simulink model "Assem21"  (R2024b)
settings: Solver=VariableStepAuto  StartTime=0.0  StopTime=5.0  RelTol=1e-3
model workspace: external: MATLAB File (data not in the file)
undefined symbols (not defined in the file or in its folder): deg, kg, Levenberg, m, Marquardt, mm, N, s, smiData, X, Y, Z
libraries: sm_lib x57, nesl_utility x7, robotcorelib x3, robotmaniplib x2
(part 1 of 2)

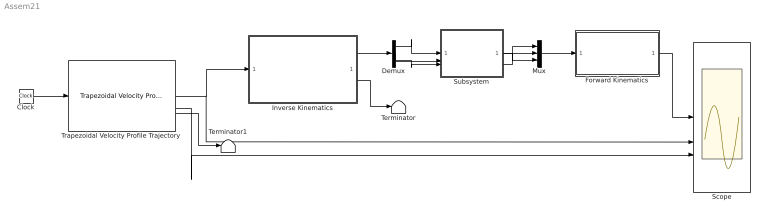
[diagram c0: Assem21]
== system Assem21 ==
  Clock : Clock
  Demux : Demux  Outputs=3
  Forward Kinematics : Subsystem
  Inverse Kinematics : Subsystem
  Mux : Mux  Inputs=3
  Scope : Scope  NumInputPorts=3
  Subsystem : Subsystem
  Terminator : Terminator
  Terminator1 : Terminator
  Trapezoidal Velocity Profile Trajectory : robotcorelib/Trapezoidal Velocity Profile Trajectory  WaypointSource=Internal  Waypoints=wp  NumParams=1  Parameter1=End Time  Parameter2=End Time  ParameterSource=Internal  PeakVelocity=[ 2; 2 ]  Acceleration=[ 1; 2 ]  EndTime=[0.5 1 1 0.5 0.5;0.5 1 1 0.5 0.5;0.5 1 1 0.5 0.5]  AccelTime=[ 1; 2 ]  SimulateUsing=Interpreted execution
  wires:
  Subsystem/2(q2m) -> Mux/2
  Subsystem/1(q1m) -> Mux/1
  Subsystem/3(q3m) -> Mux/3
  Mux/1 -> Forward Kinematics/1(Config)
  Demux/1 -> Subsystem/1(q1)
  Demux/2 -> Subsystem/2(q2)
  Demux/3 -> Subsystem/3(q3)
  Forward Kinematics/1(XYX EE) -> Scope/1
  Inverse Kinematics/1(Config) -> Demux/1
  Inverse Kinematics/2(Info) -> Terminator/1
  Clock/1 -> Trapezoidal Velocity Profile Trajectory/1
  Trapezoidal Velocity Profile Trajectory/1 -> Scope/2, Inverse Kinematics/1(In1)
  Trapezoidal Velocity Profile Trajectory/3 -> Terminator1/1
  Trapezoidal Velocity Profile Trajectory/2 -> Scope/3

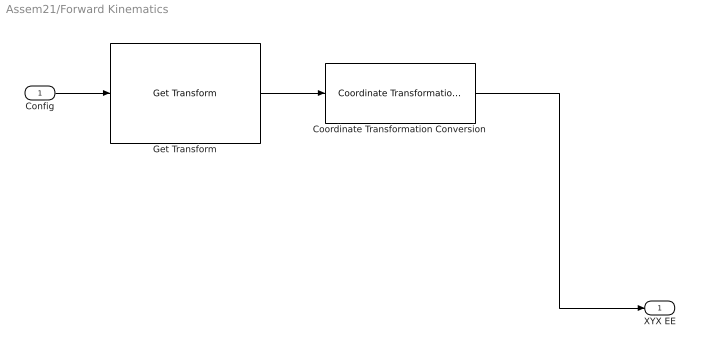
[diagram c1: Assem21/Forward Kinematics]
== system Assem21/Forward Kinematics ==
  Config : Inport
  Coordinate Transformation Conversion : robotcorelib/Coordinate Transformation Conversion  InputRepresentation=Homogeneous Transformation  InputEulerSequence=ZYX  ShowTrVecInputPort=on  OutputRepresentation=Translation Vector  OutputEulerSequence=ZYX  ShowTrVecOutputPort=on  SimulateUsing=Interpreted execution
  Get Transform : robotmaniplib/Get Transform  RigidBodyTree=DOF3_Arm  SourceBody=Body3  TargetBody=Base  SimulateUsing=Interpreted execution
  XYX EE : Outport
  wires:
  Get Transform/1 -> Coordinate Transformation Conversion/1
  Config/1 -> Get Transform/1
  Coordinate Transformation Conversion/1 -> XYX EE/1

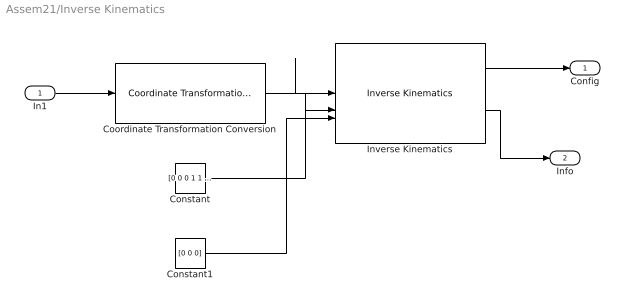
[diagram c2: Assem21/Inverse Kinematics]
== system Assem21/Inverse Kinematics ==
  In1 : Inport
  Constant : Constant  Value=[0 0 0 1 1 1]
  Constant1 : Constant  Value=[0 0 0]
  Coordinate Transformation Conversion : robotcorelib/Coordinate Transformation Conversion  InputRepresentation=Translation Vector  InputEulerSequence=ZYX  ShowTrVecInputPort=on  OutputRepresentation=Homogeneous Transformation  OutputEulerSequence=ZYX  ShowTrVecOutputPort=on  SimulateUsing=Interpreted execution
  Inverse Kinematics : robotmaniplib/Inverse Kinematics  RigidBodyTree=DOF3_Arm  EndEffector=Body3  ShowInfo=on  SolverName=Levenberg-Marquardt  EnforceJointLimits=on  MaxIterations=1500  MaxTime=10  GradientTolerance=1e-3  SolutionTolerance=1e-2  StepTolerance=1e-14  ErrorChangeTolerance=1e-3  UseErrorDamping=on  DampingBias=0.0025  SimulateUsing=Interpreted execution
  Config : Outport
  Info : Outport  Port=2
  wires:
  Constant/1 -> Inverse Kinematics/2
  In1/1 -> Coordinate Transformation Conversion/1
  Coordinate Transformation Conversion/1 -> Inverse Kinematics/1
  Inverse Kinematics/2 -> Info/1
  Inverse Kinematics/1 -> Config/1
  Constant1/1 -> Inverse Kinematics/3

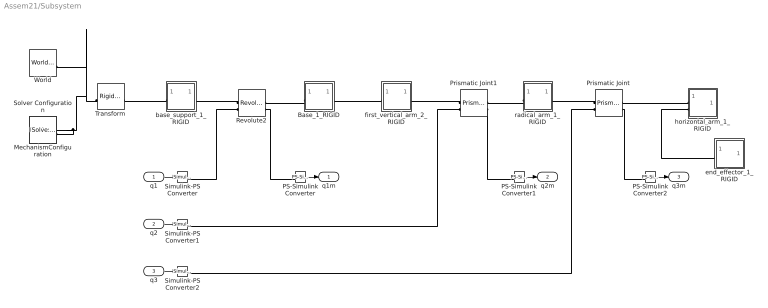
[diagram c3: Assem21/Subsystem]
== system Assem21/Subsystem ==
  q1 : Inport
  q2 : Inport  Port=2
  q3 : Inport  Port=3
  Base_1_RIGID : Subsystem
  MechanismConfiguration : sm_lib/Utilities/Mechanism Configuration  UniformGravity=Constant  GravityVector=[0 -9.80665 0]  GravityVectorUnits=m/s^2  LinearizationDelta=0.001  JointModeTransitionNonlinearIterations=2
  PS-Simulink Converter : nesl_utility/PS-Simulink Converter  PhysicalDomain=network_engine_domain  SubClassName=ps_output  LeftPortType=input  RightPortType=output  PseudoPeriodic=off  Frequencies=[]  VectorFormat=inherit  Unit=inherit  AffineConversion=off
  PS-Simulink Converter1 : nesl_utility/PS-Simulink Converter  PhysicalDomain=network_engine_domain  SubClassName=ps_output  LeftPortType=input  RightPortType=output  PseudoPeriodic=off  Frequencies=[]  VectorFormat=inherit  Unit=inherit  AffineConversion=off
  PS-Simulink Converter2 : nesl_utility/PS-Simulink Converter  PhysicalDomain=network_engine_domain  SubClassName=ps_output  LeftPortType=input  RightPortType=output  PseudoPeriodic=off  Frequencies=[]  VectorFormat=inherit  Unit=inherit  AffineConversion=off
  Prismatic Joint : sm_lib/Joints/Prismatic Joint  JointMode=Normal  CompositeWrenchDir=FollowerOnBase  CompositeWrenchFrame=BaseFrame  SenseConstraintForce=off  SenseConstraintTorque=off  SenseTotalForce=off  SenseTotalTorque=off  PositionTargetSpecify=off  PositionTargetPriority=High  PositionTargetValue=0  PositionTargetValueUnits=m  VelocityTargetSpecify=off  VelocityTargetPriority=High  VelocityTargetValue=0  VelocityTargetValueUnits=m/s  EquilibriumPosition=0  EquilibriumPositionUnits=m  SpringStiffness=0  SpringStiffnessUnits=N/m  DampingCoefficient=0  DampingCoefficientUnits=N/(m/s)  LowerLimitSpecify=on  LowerLimitBound=-1  LowerLimitBoundUnits=m  LowerLimitStiffness=1e6  LowerLimitStiffnessUnits=N/m  LowerLimitDamping=1e3  LowerLimitDampingUnits=N/(m/s)  LowerLimitTransitionRegionWidth=1e-4  LowerLimitTransitionRegionWidthUnits=m  UpperLimitSpecify=on  UpperLimitBound=1  UpperLimitBoundUnits=m  UpperLimitStiffness=1e6  UpperLimitStiffnessUnits=N/m  UpperLimitDamping=1e3  UpperLimitDampingUnits=N/(m/s)  UpperLimitTransitionRegionWidth=1e-4  UpperLimitTransitionRegionWidthUnits=m  TorqueActuationMode=ComputedTorque  MotionActuationMode=InputMotion  SensePosition=on  SenseVelocity=off  SenseAcceleration=off  SenseTorqueForce=off  SenseLowerLimitTorqueForce=off  SenseUpperLimitTorqueForce=off
  Prismatic Joint1 : sm_lib/Joints/Prismatic Joint  JointMode=Normal  CompositeWrenchDir=FollowerOnBase  CompositeWrenchFrame=BaseFrame  SenseConstraintForce=off  SenseConstraintTorque=off  SenseTotalForce=off  SenseTotalTorque=off  PositionTargetSpecify=off  PositionTargetPriority=High  PositionTargetValue=0  PositionTargetValueUnits=m  VelocityTargetSpecify=off  VelocityTargetPriority=High  VelocityTargetValue=0  VelocityTargetValueUnits=m/s  EquilibriumPosition=0  EquilibriumPositionUnits=m  SpringStiffness=0  SpringStiffnessUnits=N/m  DampingCoefficient=0  DampingCoefficientUnits=N/(m/s)  LowerLimitSpecify=on  LowerLimitBound=-1  LowerLimitBoundUnits=m  LowerLimitStiffness=1e6  LowerLimitStiffnessUnits=N/m  LowerLimitDamping=1e3  LowerLimitDampingUnits=N/(m/s)  LowerLimitTransitionRegionWidth=1e-4  LowerLimitTransitionRegionWidthUnits=m  UpperLimitSpecify=on  UpperLimitBound=1  UpperLimitBoundUnits=m  UpperLimitStiffness=1e6  UpperLimitStiffnessUnits=N/m  UpperLimitDamping=1e3  UpperLimitDampingUnits=N/(m/s)  UpperLimitTransitionRegionWidth=1e-4  UpperLimitTransitionRegionWidthUnits=m  TorqueActuationMode=ComputedTorque  MotionActuationMode=InputMotion  SensePosition=on  SenseVelocity=off  SenseAcceleration=off  SenseTorqueForce=off  SenseLowerLimitTorqueForce=off  SenseUpperLimitTorqueForce=off
  Revolute2 : sm_lib/Joints/Revolute Joint  JointMode=Normal  CompositeWrenchDir=FollowerOnBase  CompositeWrenchFrame=BaseFrame  SenseConstraintForce=off  SenseConstraintTorque=off  SenseTotalForce=off  SenseTotalTorque=off  PositionTargetSpecify=on  PositionTargetPriority=Low  PositionTargetValue=smiData.RevoluteJoint(3).Rz.Pos  PositionTargetValueUnits=deg  VelocityTargetSpecify=off  VelocityTargetPriority=High  VelocityTargetValue=0  VelocityTargetValueUnits=deg/s  EquilibriumPosition=0  EquilibriumPositionUnits=deg  SpringStiffness=0  SpringStiffnessUnits=N*m/deg  DampingCoefficient=0  DampingCoefficientUnits=N*m/(deg/s)  LowerLimitSpecify=on  LowerLimitBound=-90  LowerLimitBoundUnits=deg  LowerLimitStiffness=1e4  LowerLimitStiffnessUnits=N*m/deg  LowerLimitDamping=10  LowerLimitDampingUnits=N*m/(deg/s)  LowerLimitTransitionRegionWidth=0.1  LowerLimitTransitionRegionWidthUnits=deg  UpperLimitSpecify=on  UpperLimitBound=90  UpperLimitBoundUnits=deg  UpperLimitStiffness=1e4  UpperLimitStiffnessUnits=N*m/deg  UpperLimitDamping=10  UpperLimitDampingUnits=N*m/(deg/s)  UpperLimitTransitionRegionWidth=0.1  UpperLimitTransitionRegionWidthUnits=deg  TorqueActuationMode=ComputedTorque  MotionActuationMode=InputMotion  SensePosition=on  SenseVelocity=off  SenseAcceleration=off  SenseTorqueForce=off  SenseLowerLimitTorqueForce=off  SenseUpperLimitTorqueForce=off
  Simulink-PS Converter : nesl_utility/Simulink-PS Converter  PhysicalDomain=network_engine_domain  SubClassName=ps_input  LeftPortType=input  RightPortType=output  PseudoPeriodic=off  Frequencies=[]  NoiseDistribution=none  NoiseParameters=[]  Unit=1  AffineConversion=off  FilteringAndDerivatives=filter  SimscapeFilterOrder=2  InputFilterTimeConstant=0.001  UdotUserProvided=0
  Simulink-PS Converter1 : nesl_utility/Simulink-PS Converter  PhysicalDomain=network_engine_domain  SubClassName=ps_input  LeftPortType=input  RightPortType=output  PseudoPeriodic=off  Frequencies=[]  NoiseDistribution=none  NoiseParameters=[]  Unit=1  AffineConversion=off  FilteringAndDerivatives=filter  SimscapeFilterOrder=2  InputFilterTimeConstant=0.001  UdotUserProvided=0
  Simulink-PS Converter2 : nesl_utility/Simulink-PS Converter  PhysicalDomain=network_engine_domain  SubClassName=ps_input  LeftPortType=input  RightPortType=output  PseudoPeriodic=off  Frequencies=[]  NoiseDistribution=none  NoiseParameters=[]  Unit=1  AffineConversion=off  FilteringAndDerivatives=filter  SimscapeFilterOrder=2  InputFilterTimeConstant=0.001  UdotUserProvided=0
  Solver Configuration : nesl_utility/Solver Configuration  PhysicalDomain=network_engine_domain  SubClassName=solver  LeftPortType=input  RightPortType=generic  Tones=[]  Harmonics=[]  SimulateNoise=off  Profile=off  UseLocalSampling=off  EnableSwitchedLinearOptims=on  FrequencyDomain=off  UseCCode=off  RelTol=0.001  AbsTol=0.001  MinStep=1e-09  ToWorkspace=off  RevertToSquareIcSolve=off  NumHomotopyIterations=100  PhasorMode=off  PhasorModeNumHarmonics=1  ConsistencySolver=NEWTON_XTOL_AFTER_FTOL  IndexReductionMethod=DerivativeReplacement  DoDC=off  ResidualTolerance=1e-09  ConsistencyTolSource=GLOBAL  ConsistencyAbsTol=0.001  ConsistencyRelTol=0.001  ConsistencyTolFactor=0.001  UseLocalSolver=off  LocalSolverChoice=NE_BACKWARD_EULER_ADVANCER  ResolveIndetEquations=on  FunctionEvalNumThread=1  LocalSolverSampleTime=0.001  DoFixedCost=off  MaxNonlinIter=3  MaxModeIter=2  ComputeImpulses=off  ImpulseIterations=2  LinearAlgebra=auto  LinearAlgebraNumThread=0  EquationFormulation=NE_TIME_EF  DelaysMemoryBudget=1024  AutomaticFiltering=on  FilteringTimeConstant=0.001  PartitionStorageMethod=AS_NEEDED  PartitionMemoryBudget=1024  PartitionMethod=ROBUST  MultibodyUseLocalSolver=off  MultibodyLocalSolverChoice=ODE1  MultibodyLocalSolverSampleTime=0.001
  Transform : sm_lib/Frames and Transforms/Rigid Transform  RotationMethod=ArbitraryAxis  FollAlignAxisA=+X  BaseAlignAxisA=+Y  FollAlignAxisB=+Y  BaseAlignAxisB=+Z  RotationStandardAxis=+Z  RotationAngle=smiData.RigidTransform(21).angle  RotationAngleUnits=rad  RotationArbitraryAxis=smiData.RigidTransform(21).axis  RotationSequenceAxes=FollowerAxes  RotationSequence=XYX  RotationSequenceAngles=[0 0 0]  RotationSequenceAnglesUnits=deg  RotationMatrix=[1 0 0;0 1 0;0 0 1]  Quaternion=[1 0 0 0]  TranslationMethod=Cartesian  TranslationCartesianOffset=smiData.RigidTransform(21).translation  TranslationCartesianOffsetUnits=mm  TranslationStandardAxis=+Z  TranslationStandardOffset=0  TranslationStandardOffsetUnits=m  TranslationROffset=0  TranslationROffsetUnits=m  TranslationThetaOffset=0  TranslationThetaOffsetUnits=deg  TranslationZOffset=0  TranslationZOffsetUnits=m
  World : sm_lib/Frames and Transforms/World Frame
  base_support_1_RIGID : Subsystem
  end_effector_1_RIGID : Subsystem
  first_vertical_arm_2_RIGID : Subsystem
  horizontal_arm_1_RIGID : Subsystem
  radical_arm_1_RIGID : Subsystem
  q1m : Outport
  q2m : Outport  Port=2
  q3m : Outport  Port=3
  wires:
  q2/1 -> Simulink-PS Converter1/1
  PS-Simulink Converter1/1 -> q2m/1
  PS-Simulink Converter/1 -> q1m/1
  q3/1 -> Simulink-PS Converter2/1
  PS-Simulink Converter2/1 -> q3m/1
  q1/1 -> Simulink-PS Converter/1
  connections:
  Transform/LConn1 -- MechanismConfiguration/RConn1 -- Solver Configuration/RConn1 -- World/RConn1
  Base_1_RIGID/LConn1 -- Revolute2/RConn1
  end_effector_1_RIGID/LConn1 -- horizontal_arm_1_RIGID/LConn2
  Prismatic Joint1/LConn1 -- first_vertical_arm_2_RIGID/RConn1
  Revolute2/RConn2 -- PS-Simulink Converter/LConn1
  Revolute2/LConn1 -- base_support_1_RIGID/RConn1
  Base_1_RIGID/RConn1 -- first_vertical_arm_2_RIGID/LConn1
  Transform/RConn1 -- base_support_1_RIGID/LConn1
  Prismatic Joint/LConn1 -- radical_arm_1_RIGID/RConn1
  horizontal_arm_1_RIGID/LConn1 -- Prismatic Joint/RConn1
  radical_arm_1_RIGID/LConn1 -- Prismatic Joint1/RConn1
  Prismatic Joint/RConn2 -- PS-Simulink Converter2/LConn1
  Simulink-PS Converter2/RConn1 -- Prismatic Joint/LConn2
  Prismatic Joint1/RConn2 -- PS-Simulink Converter1/LConn1
  Simulink-PS Converter/RConn1 -- Revolute2/LConn2
  Simulink-PS Converter1/RConn1 -- Prismatic Joint1/LConn2

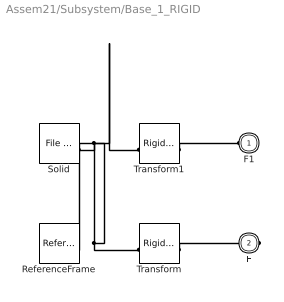
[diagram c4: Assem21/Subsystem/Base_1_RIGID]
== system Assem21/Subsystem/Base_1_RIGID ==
  ReferenceFrame : sm_lib/Frames and Transforms/Reference Frame
  Solid : sm_lib/Body Elements/File Solid  ExtGeomFileName=Base_Default_sldprt.STEP  UnitType=FromFile  ExtGeomFileUnits=m  StepReaderType=HEX  ExportConvexHullGeometry=off  InertiaType=Custom  BasedOnType=DensityFromFile  Density=1000  DensityUnits=kg/m^3  Mass=smiData.Solid(8).mass  MassUnits=kg  CenterOfMass=smiData.Solid(8).CoM  CenterOfMassUnits=mm  MomentsOfInertia=smiData.Solid(8).MoI  MomentsOfInertiaUnits=kg*mm^2  ProductsOfInertia=smiData.Solid(8).PoI  ProductsOfInertiaUnits=kg*mm^2  GraphicType=FromGeometry  MarkerShape=Sphere  MarkerSize=10  GraphicVisPropType=SimpleVisualProperties  GraphicDiffuseColor=smiData.Solid(8).color  GraphicOpacity=smiData.Solid(8).opacity  GraphicSpecularColor=[0.5 0.5 0.5 1.0]  GraphicAmbientColor=[0.15 0.15 0.15 1.0]  GraphicEmissiveColor=[0.0 0.0 0.0 1.0]  GraphicShininess=75  DoExposeReferenceFrame=on  SerializedFrames=<Frames/>
  Transform : sm_lib/Frames and Transforms/Rigid Transform  RotationMethod=ArbitraryAxis  FollAlignAxisA=+X  BaseAlignAxisA=+Y  FollAlignAxisB=+Y  BaseAlignAxisB=+Z  RotationStandardAxis=+Z  RotationAngle=smiData.RigidTransform(5).angle  RotationAngleUnits=rad  RotationArbitraryAxis=smiData.RigidTransform(5).axis  RotationSequenceAxes=FollowerAxes  RotationSequence=XYX  RotationSequenceAngles=[0 0 0]  RotationSequenceAnglesUnits=deg  RotationMatrix=[1 0 0;0 1 0;0 0 1]  Quaternion=[1 0 0 0]  TranslationMethod=Cartesian  TranslationCartesianOffset=smiData.RigidTransform(5).translation  TranslationCartesianOffsetUnits=mm  TranslationStandardAxis=+Z  TranslationStandardOffset=0  TranslationStandardOffsetUnits=m  TranslationROffset=0  TranslationROffsetUnits=m  TranslationThetaOffset=0  TranslationThetaOffsetUnits=deg  TranslationZOffset=0  TranslationZOffsetUnits=m
  Transform1 : sm_lib/Frames and Transforms/Rigid Transform  RotationMethod=ArbitraryAxis  FollAlignAxisA=+X  BaseAlignAxisA=+Y  FollAlignAxisB=+Y  BaseAlignAxisB=+Z  RotationStandardAxis=+Z  RotationAngle=smiData.RigidTransform(10).angle  RotationAngleUnits=rad  RotationArbitraryAxis=smiData.RigidTransform(10).axis  RotationSequenceAxes=FollowerAxes  RotationSequence=XYX  RotationSequenceAngles=[0 0 0]  RotationSequenceAnglesUnits=deg  RotationMatrix=[1 0 0;0 1 0;0 0 1]  Quaternion=[1 0 0 0]  TranslationMethod=Cartesian  TranslationCartesianOffset=smiData.RigidTransform(10).translation  TranslationCartesianOffsetUnits=mm  TranslationStandardAxis=+Z  TranslationStandardOffset=0  TranslationStandardOffsetUnits=m  TranslationROffset=0  TranslationROffsetUnits=m  TranslationThetaOffset=0  TranslationThetaOffsetUnits=deg  TranslationZOffset=0  TranslationZOffsetUnits=m
  F1 : PMIOPort  Side=Left
  F : PMIOPort  Port=2  Side=Right
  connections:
  Solid/RConn1 -- ReferenceFrame/RConn1 -- Transform/LConn1 -- Transform1/LConn1
  Transform/RConn1 -- F/RConn1
  Transform1/RConn1 -- F1/RConn1

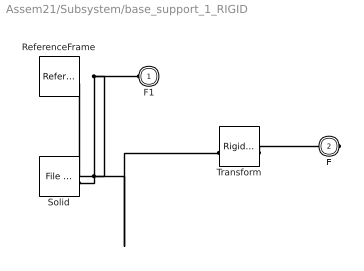
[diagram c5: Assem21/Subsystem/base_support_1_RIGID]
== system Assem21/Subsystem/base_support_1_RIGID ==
  ReferenceFrame : sm_lib/Frames and Transforms/Reference Frame
  Solid : sm_lib/Body Elements/File Solid  ExtGeomFileName=base support_Default_sldprt.STEP  UnitType=FromFile  ExtGeomFileUnits=m  StepReaderType=HEX  ExportConvexHullGeometry=off  InertiaType=Custom  BasedOnType=DensityFromFile  Density=1000  DensityUnits=kg/m^3  Mass=smiData.Solid(9).mass  MassUnits=kg  CenterOfMass=smiData.Solid(9).CoM  CenterOfMassUnits=mm  MomentsOfInertia=smiData.Solid(9).MoI  MomentsOfInertiaUnits=kg*mm^2  ProductsOfInertia=smiData.Solid(9).PoI  ProductsOfInertiaUnits=kg*mm^2  GraphicType=FromGeometry  MarkerShape=Sphere  MarkerSize=10  GraphicVisPropType=SimpleVisualProperties  GraphicDiffuseColor=smiData.Solid(9).color  GraphicOpacity=smiData.Solid(9).opacity  GraphicSpecularColor=[0.5 0.5 0.5 1.0]  GraphicAmbientColor=[0.15 0.15 0.15 1.0]  GraphicEmissiveColor=[0.0 0.0 0.0 1.0]  GraphicShininess=75  DoExposeReferenceFrame=on  SerializedFrames=<Frames/>
  Transform : sm_lib/Frames and Transforms/Rigid Transform  RotationMethod=ArbitraryAxis  FollAlignAxisA=+X  BaseAlignAxisA=+Y  FollAlignAxisB=+Y  BaseAlignAxisB=+Z  RotationStandardAxis=+Z  RotationAngle=smiData.RigidTransform(9).angle  RotationAngleUnits=rad  RotationArbitraryAxis=smiData.RigidTransform(9).axis  RotationSequenceAxes=FollowerAxes  RotationSequence=XYX  RotationSequenceAngles=[0 0 0]  RotationSequenceAnglesUnits=deg  RotationMatrix=[1 0 0;0 1 0;0 0 1]  Quaternion=[1 0 0 0]  TranslationMethod=Cartesian  TranslationCartesianOffset=smiData.RigidTransform(9).translation  TranslationCartesianOffsetUnits=mm  TranslationStandardAxis=+Z  TranslationStandardOffset=0  TranslationStandardOffsetUnits=m  TranslationROffset=0  TranslationROffsetUnits=m  TranslationThetaOffset=0  TranslationThetaOffsetUnits=deg  TranslationZOffset=0  TranslationZOffsetUnits=m
  F1 : PMIOPort  Side=Left
  F : PMIOPort  Port=2  Side=Right
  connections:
  Solid/RConn1 -- ReferenceFrame/RConn1 -- Transform/LConn1 -- F1/RConn1
  Transform/RConn1 -- F/RConn1

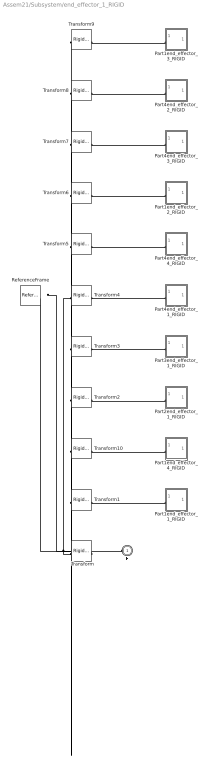
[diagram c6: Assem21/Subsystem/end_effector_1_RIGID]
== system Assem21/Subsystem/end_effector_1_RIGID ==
  Part1end_effector_1_RIGID : Subsystem
  Part1end_effector_2_RIGID : Subsystem
  Part1end_effector_3_RIGID : Subsystem
  Part1end_effector_4_RIGID : Subsystem
  Part2end_effector_1_RIGID : Subsystem
  Part3end_effector_1_RIGID : Subsystem
  Part4end_effector_1_RIGID : Subsystem
  Part4end_effector_2_RIGID : Subsystem
  Part4end_effector_3_RIGID : Subsystem
  Part4end_effector_4_RIGID : Subsystem
  ReferenceFrame : sm_lib/Frames and Transforms/Reference Frame
  Transform : sm_lib/Frames and Transforms/Rigid Transform  RotationMethod=ArbitraryAxis  FollAlignAxisA=+X  BaseAlignAxisA=+Y  FollAlignAxisB=+Y  BaseAlignAxisB=+Z  RotationStandardAxis=+Z  RotationAngle=smiData.RigidTransform(2).angle  RotationAngleUnits=rad  RotationArbitraryAxis=smiData.RigidTransform(2).axis  RotationSequenceAxes=FollowerAxes  RotationSequence=XYX  RotationSequenceAngles=[0 0 0]  RotationSequenceAnglesUnits=deg  RotationMatrix=[1 0 0;0 1 0;0 0 1]  Quaternion=[1 0 0 0]  TranslationMethod=Cartesian  TranslationCartesianOffset=smiData.RigidTransform(2).translation  TranslationCartesianOffsetUnits=mm  TranslationStandardAxis=+Z  TranslationStandardOffset=0  TranslationStandardOffsetUnits=m  TranslationROffset=0  TranslationROffsetUnits=m  TranslationThetaOffset=0  TranslationThetaOffsetUnits=deg  TranslationZOffset=0  TranslationZOffsetUnits=m
  Transform1 : sm_lib/Frames and Transforms/Rigid Transform  RotationMethod=ArbitraryAxis  FollAlignAxisA=+X  BaseAlignAxisA=+Y  FollAlignAxisB=+Y  BaseAlignAxisB=+Z  RotationStandardAxis=+Z  RotationAngle=smiData.RigidTransform(11).angle  RotationAngleUnits=rad  RotationArbitraryAxis=smiData.RigidTransform(11).axis  RotationSequenceAxes=FollowerAxes  RotationSequence=XYX  RotationSequenceAngles=[0 0 0]  RotationSequenceAnglesUnits=deg  RotationMatrix=[1 0 0;0 1 0;0 0 1]  Quaternion=[1 0 0 0]  TranslationMethod=Cartesian  TranslationCartesianOffset=smiData.RigidTransform(11).translation  TranslationCartesianOffsetUnits=mm  TranslationStandardAxis=+Z  TranslationStandardOffset=0  TranslationStandardOffsetUnits=m  TranslationROffset=0  TranslationROffsetUnits=m  TranslationThetaOffset=0  TranslationThetaOffsetUnits=deg  TranslationZOffset=0  TranslationZOffsetUnits=m
  Transform10 : sm_lib/Frames and Transforms/Rigid Transform  RotationMethod=ArbitraryAxis  FollAlignAxisA=+X  BaseAlignAxisA=+Y  FollAlignAxisB=+Y  BaseAlignAxisB=+Z  RotationStandardAxis=+Z  RotationAngle=smiData.RigidTransform(20).angle  RotationAngleUnits=rad  RotationArbitraryAxis=smiData.RigidTransform(20).axis  RotationSequenceAxes=FollowerAxes  RotationSequence=XYX  RotationSequenceAngles=[0 0 0]  RotationSequenceAnglesUnits=deg  RotationMatrix=[1 0 0;0 1 0;0 0 1]  Quaternion=[1 0 0 0]  TranslationMethod=Cartesian  TranslationCartesianOffset=smiData.RigidTransform(20).translation  TranslationCartesianOffsetUnits=mm  TranslationStandardAxis=+Z  TranslationStandardOffset=0  TranslationStandardOffsetUnits=m  TranslationROffset=0  TranslationROffsetUnits=m  TranslationThetaOffset=0  TranslationThetaOffsetUnits=deg  TranslationZOffset=0  TranslationZOffsetUnits=m
  Transform2 : sm_lib/Frames and Transforms/Rigid Transform  RotationMethod=ArbitraryAxis  FollAlignAxisA=+X  BaseAlignAxisA=+Y  FollAlignAxisB=+Y  BaseAlignAxisB=+Z  RotationStandardAxis=+Z  RotationAngle=smiData.RigidTransform(12).angle  RotationAngleUnits=rad  RotationArbitraryAxis=smiData.RigidTransform(12).axis  RotationSequenceAxes=FollowerAxes  RotationSequence=XYX  RotationSequenceAngles=[0 0 0]  RotationSequenceAnglesUnits=deg  RotationMatrix=[1 0 0;0 1 0;0 0 1]  Quaternion=[1 0 0 0]  TranslationMethod=Cartesian  TranslationCartesianOffset=smiData.RigidTransform(12).translation  TranslationCartesianOffsetUnits=mm  TranslationStandardAxis=+Z  TranslationStandardOffset=0  TranslationStandardOffsetUnits=m  TranslationROffset=0  TranslationROffsetUnits=m  TranslationThetaOffset=0  TranslationThetaOffsetUnits=deg  TranslationZOffset=0  TranslationZOffsetUnits=m
  Transform3 : sm_lib/Frames and Transforms/Rigid Transform  RotationMethod=ArbitraryAxis  FollAlignAxisA=+X  BaseAlignAxisA=+Y  FollAlignAxisB=+Y  BaseAlignAxisB=+Z  RotationStandardAxis=+Z  RotationAngle=smiData.RigidTransform(13).angle  RotationAngleUnits=rad  RotationArbitraryAxis=smiData.RigidTransform(13).axis  RotationSequenceAxes=FollowerAxes  RotationSequence=XYX  RotationSequenceAngles=[0 0 0]  RotationSequenceAnglesUnits=deg  RotationMatrix=[1 0 0;0 1 0;0 0 1]  Quaternion=[1 0 0 0]  TranslationMethod=Cartesian  TranslationCartesianOffset=smiData.RigidTransform(13).translation  TranslationCartesianOffsetUnits=mm  TranslationStandardAxis=+Z  TranslationStandardOffset=0  TranslationStandardOffsetUnits=m  TranslationROffset=0  TranslationROffsetUnits=m  TranslationThetaOffset=0  TranslationThetaOffsetUnits=deg  TranslationZOffset=0  TranslationZOffsetUnits=m
  Transform4 : sm_lib/Frames and Transforms/Rigid Transform  RotationMethod=ArbitraryAxis  FollAlignAxisA=+X  BaseAlignAxisA=+Y  FollAlignAxisB=+Y  BaseAlignAxisB=+Z  RotationStandardAxis=+Z  RotationAngle=smiData.RigidTransform(14).angle  RotationAngleUnits=rad  RotationArbitraryAxis=smiData.RigidTransform(14).axis  RotationSequenceAxes=FollowerAxes  RotationSequence=XYX  RotationSequenceAngles=[0 0 0]  RotationSequenceAnglesUnits=deg  RotationMatrix=[1 0 0;0 1 0;0 0 1]  Quaternion=[1 0 0 0]  TranslationMethod=Cartesian  TranslationCartesianOffset=smiData.RigidTransform(14).translation  TranslationCartesianOffsetUnits=mm  TranslationStandardAxis=+Z  TranslationStandardOffset=0  TranslationStandardOffsetUnits=m  TranslationROffset=0  TranslationROffsetUnits=m  TranslationThetaOffset=0  TranslationThetaOffsetUnits=deg  TranslationZOffset=0  TranslationZOffsetUnits=m
  Transform5 : sm_lib/Frames and Transforms/Rigid Transform  RotationMethod=ArbitraryAxis  FollAlignAxisA=+X  BaseAlignAxisA=+Y  FollAlignAxisB=+Y  BaseAlignAxisB=+Z  RotationStandardAxis=+Z  RotationAngle=smiData.RigidTransform(15).angle  RotationAngleUnits=rad  RotationArbitraryAxis=smiData.RigidTransform(15).axis  RotationSequenceAxes=FollowerAxes  RotationSequence=XYX  RotationSequenceAngles=[0 0 0]  RotationSequenceAnglesUnits=deg  RotationMatrix=[1 0 0;0 1 0;0 0 1]  Quaternion=[1 0 0 0]  TranslationMethod=Cartesian  TranslationCartesianOffset=smiData.RigidTransform(15).translation  TranslationCartesianOffsetUnits=mm  TranslationStandardAxis=+Z  TranslationStandardOffset=0  TranslationStandardOffsetUnits=m  TranslationROffset=0  TranslationROffsetUnits=m  TranslationThetaOffset=0  TranslationThetaOffsetUnits=deg  TranslationZOffset=0  TranslationZOffsetUnits=m
  Transform6 : sm_lib/Frames and Transforms/Rigid Transform  RotationMethod=ArbitraryAxis  FollAlignAxisA=+X  BaseAlignAxisA=+Y  FollAlignAxisB=+Y  BaseAlignAxisB=+Z  RotationStandardAxis=+Z  RotationAngle=smiData.RigidTransform(16).angle  RotationAngleUnits=rad  RotationArbitraryAxis=smiData.RigidTransform(16).axis  RotationSequenceAxes=FollowerAxes  RotationSequence=XYX  RotationSequenceAngles=[0 0 0]  RotationSequenceAnglesUnits=deg  RotationMatrix=[1 0 0;0 1 0;0 0 1]  Quaternion=[1 0 0 0]  TranslationMethod=Cartesian  TranslationCartesianOffset=smiData.RigidTransform(16).translation  TranslationCartesianOffsetUnits=mm  TranslationStandardAxis=+Z  TranslationStandardOffset=0  TranslationStandardOffsetUnits=m  TranslationROffset=0  TranslationROffsetUnits=m  TranslationThetaOffset=0  TranslationThetaOffsetUnits=deg  TranslationZOffset=0  TranslationZOffsetUnits=m
  Transform7 : sm_lib/Frames and Transforms/Rigid Transform  RotationMethod=ArbitraryAxis  FollAlignAxisA=+X  BaseAlignAxisA=+Y  FollAlignAxisB=+Y  BaseAlignAxisB=+Z  RotationStandardAxis=+Z  RotationAngle=smiData.RigidTransform(17).angle  RotationAngleUnits=rad  RotationArbitraryAxis=smiData.RigidTransform(17).axis  RotationSequenceAxes=FollowerAxes  RotationSequence=XYX  RotationSequenceAngles=[0 0 0]  RotationSequenceAnglesUnits=deg  RotationMatrix=[1 0 0;0 1 0;0 0 1]  Quaternion=[1 0 0 0]  TranslationMethod=Cartesian  TranslationCartesianOffset=smiData.RigidTransform(17).translation  TranslationCartesianOffsetUnits=mm  TranslationStandardAxis=+Z  TranslationStandardOffset=0  TranslationStandardOffsetUnits=m  TranslationROffset=0  TranslationROffsetUnits=m  TranslationThetaOffset=0  TranslationThetaOffsetUnits=deg  TranslationZOffset=0  TranslationZOffsetUnits=m
  Transform8 : sm_lib/Frames and Transforms/Rigid Transform  RotationMethod=ArbitraryAxis  FollAlignAxisA=+X  BaseAlignAxisA=+Y  FollAlignAxisB=+Y  BaseAlignAxisB=+Z  RotationStandardAxis=+Z  RotationAngle=smiData.RigidTransform(18).angle  RotationAngleUnits=rad  RotationArbitraryAxis=smiData.RigidTransform(18).axis  RotationSequenceAxes=FollowerAxes  RotationSequence=XYX  RotationSequenceAngles=[0 0 0]  RotationSequenceAnglesUnits=deg  RotationMatrix=[1 0 0;0 1 0;0 0 1]  Quaternion=[1 0 0 0]  TranslationMethod=Cartesian  TranslationCartesianOffset=smiData.RigidTransform(18).translation  TranslationCartesianOffsetUnits=mm  TranslationStandardAxis=+Z  TranslationStandardOffset=0  TranslationStandardOffsetUnits=m  TranslationROffset=0  TranslationROffsetUnits=m  TranslationThetaOffset=0  TranslationThetaOffsetUnits=deg  TranslationZOffset=0  TranslationZOffsetUnits=m
  Transform9 : sm_lib/Frames and Transforms/Rigid Transform  RotationMethod=ArbitraryAxis  FollAlignAxisA=+X  BaseAlignAxisA=+Y  FollAlignAxisB=+Y  BaseAlignAxisB=+Z  RotationStandardAxis=+Z  RotationAngle=smiData.RigidTransform(19).angle  RotationAngleUnits=rad  RotationArbitraryAxis=smiData.RigidTransform(19).axis  RotationSequenceAxes=FollowerAxes  RotationSequence=XYX  RotationSequenceAngles=[0 0 0]  RotationSequenceAnglesUnits=deg  RotationMatrix=[1 0 0;0 1 0;0 0 1]  Quaternion=[1 0 0 0]  TranslationMethod=Cartesian  TranslationCartesianOffset=smiData.RigidTransform(19).translation  TranslationCartesianOffsetUnits=mm  TranslationStandardAxis=+Z  TranslationStandardOffset=0  TranslationStandardOffsetUnits=m  TranslationROffset=0  TranslationROffsetUnits=m  TranslationThetaOffset=0  TranslationThetaOffsetUnits=deg  TranslationZOffset=0  TranslationZOffsetUnits=m
  F : PMIOPort  Side=Left
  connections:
  Transform/LConn1 -- ReferenceFrame/RConn1 -- Transform1/LConn1 -- Transform10/LConn1 -- Transform2/LConn1 -- Transform3/LConn1 -- Transform4/LConn1 -- Transform5/LConn1 -- Transform6/LConn1 -- Transform7/LConn1 -- Transform8/LConn1 -- Transform9/LConn1
  Transform/RConn1 -- F/RConn1
  Part1end_effector_3_RIGID/LConn1 -- Transform9/RConn1
  Part1end_effector_4_RIGID/LConn1 -- Transform10/RConn1
  Part1end_effector_1_RIGID/LConn1 -- Transform1/RConn1
  Part2end_effector_1_RIGID/LConn1 -- Transform2/RConn1
  Part3end_effector_1_RIGID/LConn1 -- Transform3/RConn1
  Part4end_effector_1_RIGID/LConn1 -- Transform4/RConn1
  Part4end_effector_4_RIGID/LConn1 -- Transform5/RConn1
  Part1end_effector_2_RIGID/LConn1 -- Transform6/RConn1
  Part4end_effector_3_RIGID/LConn1 -- Transform7/RConn1
  Part4end_effector_2_RIGID/LConn1 -- Transform8/RConn1

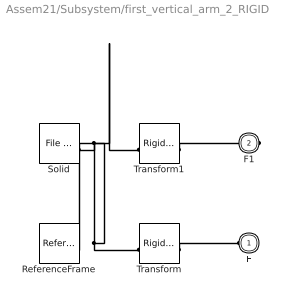
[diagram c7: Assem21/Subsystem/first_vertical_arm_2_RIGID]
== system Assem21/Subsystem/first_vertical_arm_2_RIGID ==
  ReferenceFrame : sm_lib/Frames and Transforms/Reference Frame
  Solid : sm_lib/Body Elements/File Solid  ExtGeomFileName=first vertical arm_Default_sldprt.STEP  UnitType=FromFile  ExtGeomFileUnits=m  StepReaderType=HEX  ExportConvexHullGeometry=off  InertiaType=Custom  BasedOnType=DensityFromFile  Density=1000  DensityUnits=kg/m^3  Mass=smiData.Solid(3).mass  MassUnits=kg  CenterOfMass=smiData.Solid(3).CoM  CenterOfMassUnits=mm  MomentsOfInertia=smiData.Solid(3).MoI  MomentsOfInertiaUnits=kg*mm^2  ProductsOfInertia=smiData.Solid(3).PoI  ProductsOfInertiaUnits=kg*mm^2  GraphicType=FromGeometry  MarkerShape=Sphere  MarkerSize=10  GraphicVisPropType=SimpleVisualProperties  GraphicDiffuseColor=smiData.Solid(3).color  GraphicOpacity=smiData.Solid(3).opacity  GraphicSpecularColor=[0.5 0.5 0.5 1.0]  GraphicAmbientColor=[0.15 0.15 0.15 1.0]  GraphicEmissiveColor=[0.0 0.0 0.0 1.0]  GraphicShininess=75  DoExposeReferenceFrame=on  SerializedFrames=<Frames/>
  Transform : sm_lib/Frames and Transforms/Rigid Transform  RotationMethod=ArbitraryAxis  FollAlignAxisA=+X  BaseAlignAxisA=+Y  FollAlignAxisB=+Y  BaseAlignAxisB=+Z  RotationStandardAxis=+Z  RotationAngle=smiData.RigidTransform(6).angle  RotationAngleUnits=rad  RotationArbitraryAxis=smiData.RigidTransform(6).axis  RotationSequenceAxes=FollowerAxes  RotationSequence=XYX  RotationSequenceAngles=[0 0 0]  RotationSequenceAnglesUnits=deg  RotationMatrix=[1 0 0;0 1 0;0 0 1]  Quaternion=[1 0 0 0]  TranslationMethod=Cartesian  TranslationCartesianOffset=smiData.RigidTransform(6).translation  TranslationCartesianOffsetUnits=mm  TranslationStandardAxis=+Z  TranslationStandardOffset=0  TranslationStandardOffsetUnits=m  TranslationROffset=0  TranslationROffsetUnits=m  TranslationThetaOffset=0  TranslationThetaOffsetUnits=deg  TranslationZOffset=0  TranslationZOffsetUnits=m
  Transform1 : sm_lib/Frames and Transforms/Rigid Transform  RotationMethod=ArbitraryAxis  FollAlignAxisA=+X  BaseAlignAxisA=+Y  FollAlignAxisB=+Y  BaseAlignAxisB=+Z  RotationStandardAxis=+Z  RotationAngle=smiData.RigidTransform(7).angle  RotationAngleUnits=rad  RotationArbitraryAxis=smiData.RigidTransform(7).axis  RotationSequenceAxes=FollowerAxes  RotationSequence=XYX  RotationSequenceAngles=[0 0 0]  RotationSequenceAnglesUnits=deg  RotationMatrix=[1 0 0;0 1 0;0 0 1]  Quaternion=[1 0 0 0]  TranslationMethod=Cartesian  TranslationCartesianOffset=smiData.RigidTransform(7).translation  TranslationCartesianOffsetUnits=mm  TranslationStandardAxis=+Z  TranslationStandardOffset=0  TranslationStandardOffsetUnits=m  TranslationROffset=0  TranslationROffsetUnits=m  TranslationThetaOffset=0  TranslationThetaOffsetUnits=deg  TranslationZOffset=0  TranslationZOffsetUnits=m
  F : PMIOPort  Side=Left
  F1 : PMIOPort  Port=2  Side=Right
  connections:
  Solid/RConn1 -- ReferenceFrame/RConn1 -- Transform/LConn1 -- Transform1/LConn1
  Transform/RConn1 -- F/RConn1
  Transform1/RConn1 -- F1/RConn1

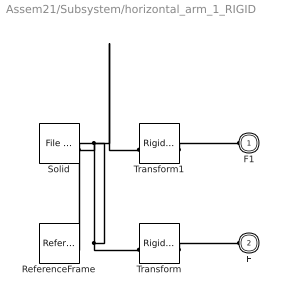
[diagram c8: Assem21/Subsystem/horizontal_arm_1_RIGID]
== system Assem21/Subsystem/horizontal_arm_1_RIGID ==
  ReferenceFrame : sm_lib/Frames and Transforms/Reference Frame
  Solid : sm_lib/Body Elements/File Solid  ExtGeomFileName=horizontal arm_Default_sldprt.STEP  UnitType=FromFile  ExtGeomFileUnits=m  StepReaderType=HEX  ExportConvexHullGeometry=off  InertiaType=Custom  BasedOnType=DensityFromFile  Density=1000  DensityUnits=kg/m^3  Mass=smiData.Solid(2).mass  MassUnits=kg  CenterOfMass=smiData.Solid(2).CoM  CenterOfMassUnits=mm  MomentsOfInertia=smiData.Solid(2).MoI  MomentsOfInertiaUnits=kg*mm^2  ProductsOfInertia=smiData.Solid(2).PoI  ProductsOfInertiaUnits=kg*mm^2  GraphicType=FromGeometry  MarkerShape=Sphere  MarkerSize=10  GraphicVisPropType=SimpleVisualProperties  GraphicDiffuseColor=smiData.Solid(2).color  GraphicOpacity=smiData.Solid(2).opacity  GraphicSpecularColor=[0.5 0.5 0.5 1.0]  GraphicAmbientColor=[0.15 0.15 0.15 1.0]  GraphicEmissiveColor=[0.0 0.0 0.0 1.0]  GraphicShininess=75  DoExposeReferenceFrame=on  SerializedFrames=<Frames/>
  Transform : sm_lib/Frames and Transforms/Rigid Transform  RotationMethod=ArbitraryAxis  FollAlignAxisA=+X  BaseAlignAxisA=+Y  FollAlignAxisB=+Y  BaseAlignAxisB=+Z  RotationStandardAxis=+Z  RotationAngle=smiData.RigidTransform(1).angle  RotationAngleUnits=rad  RotationArbitraryAxis=smiData.RigidTransform(1).axis  RotationSequenceAxes=FollowerAxes  RotationSequence=XYX  RotationSequenceAngles=[0 0 0]  RotationSequenceAnglesUnits=deg  RotationMatrix=[1 0 0;0 1 0;0 0 1]  Quaternion=[1 0 0 0]  TranslationMethod=Cartesian  TranslationCartesianOffset=smiData.RigidTransform(1).translation  TranslationCartesianOffsetUnits=mm  TranslationStandardAxis=+Z  TranslationStandardOffset=0  TranslationStandardOffsetUnits=m  TranslationROffset=0  TranslationROffsetUnits=m  TranslationThetaOffset=0  TranslationThetaOffsetUnits=deg  TranslationZOffset=0  TranslationZOffsetUnits=m
  Transform1 : sm_lib/Frames and Transforms/Rigid Transform  RotationMethod=ArbitraryAxis  FollAlignAxisA=+X  BaseAlignAxisA=+Y  FollAlignAxisB=+Y  BaseAlignAxisB=+Z  RotationStandardAxis=+Z  RotationAngle=smiData.RigidTransform(4).angle  RotationAngleUnits=rad  RotationArbitraryAxis=smiData.RigidTransform(4).axis  RotationSequenceAxes=FollowerAxes  RotationSequence=XYX  RotationSequenceAngles=[0 0 0]  RotationSequenceAnglesUnits=deg  RotationMatrix=[1 0 0;0 1 0;0 0 1]  Quaternion=[1 0 0 0]  TranslationMethod=Cartesian  TranslationCartesianOffset=smiData.RigidTransform(4).translation  TranslationCartesianOffsetUnits=mm  TranslationStandardAxis=+Z  TranslationStandardOffset=0  TranslationStandardOffsetUnits=m  TranslationROffset=0  TranslationROffsetUnits=m  TranslationThetaOffset=0  TranslationThetaOffsetUnits=deg  TranslationZOffset=0  TranslationZOffsetUnits=m
  F1 : PMIOPort  Side=Left
  F : PMIOPort  Port=2  Side=Left
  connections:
  Solid/RConn1 -- ReferenceFrame/RConn1 -- Transform/LConn1 -- Transform1/LConn1
  Transform/RConn1 -- F/RConn1
  Transform1/RConn1 -- F1/RConn1

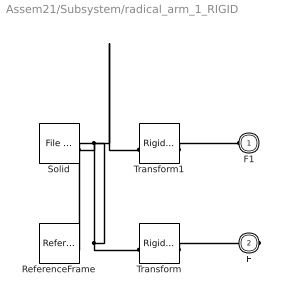
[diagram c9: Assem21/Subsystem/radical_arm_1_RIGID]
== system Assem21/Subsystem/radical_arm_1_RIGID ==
  ReferenceFrame : sm_lib/Frames and Transforms/Reference Frame
  Solid : sm_lib/Body Elements/File Solid  ExtGeomFileName=radical arm_Default_sldprt.STEP  UnitType=FromFile  ExtGeomFileUnits=m  StepReaderType=HEX  ExportConvexHullGeometry=off  InertiaType=Custom  BasedOnType=DensityFromFile  Density=1000  DensityUnits=kg/m^3  Mass=smiData.Solid(1).mass  MassUnits=kg  CenterOfMass=smiData.Solid(1).CoM  CenterOfMassUnits=mm  MomentsOfInertia=smiData.Solid(1).MoI  MomentsOfInertiaUnits=kg*mm^2  ProductsOfInertia=smiData.Solid(1).PoI  ProductsOfInertiaUnits=kg*mm^2  GraphicType=FromGeometry  MarkerShape=Sphere  MarkerSize=10  GraphicVisPropType=SimpleVisualProperties  GraphicDiffuseColor=smiData.Solid(1).color  GraphicOpacity=smiData.Solid(1).opacity  GraphicSpecularColor=[0.5 0.5 0.5 1.0]  GraphicAmbientColor=[0.15 0.15 0.15 1.0]  GraphicEmissiveColor=[0.0 0.0 0.0 1.0]  GraphicShininess=75  DoExposeReferenceFrame=on  SerializedFrames=<Frames/>
  Transform : sm_lib/Frames and Transforms/Rigid Transform  RotationMethod=ArbitraryAxis  FollAlignAxisA=+X  BaseAlignAxisA=+Y  FollAlignAxisB=+Y  BaseAlignAxisB=+Z  RotationStandardAxis=+Z  RotationAngle=smiData.RigidTransform(3).angle  RotationAngleUnits=rad  RotationArbitraryAxis=smiData.RigidTransform(3).axis  RotationSequenceAxes=FollowerAxes  RotationSequence=XYX  RotationSequenceAngles=[0 0 0]  RotationSequenceAnglesUnits=deg  RotationMatrix=[1 0 0;0 1 0;0 0 1]  Quaternion=[1 0 0 0]  TranslationMethod=Cartesian  TranslationCartesianOffset=smiData.RigidTransform(3).translation  TranslationCartesianOffsetUnits=mm  TranslationStandardAxis=+Z  TranslationStandardOffset=0  TranslationStandardOffsetUnits=m  TranslationROffset=0  TranslationROffsetUnits=m  TranslationThetaOffset=0  TranslationThetaOffsetUnits=deg  TranslationZOffset=0  TranslationZOffsetUnits=m
  Transform1 : sm_lib/Frames and Transforms/Rigid Transform  RotationMethod=ArbitraryAxis  FollAlignAxisA=+X  BaseAlignAxisA=+Y  FollAlignAxisB=+Y  BaseAlignAxisB=+Z  RotationStandardAxis=+Z  RotationAngle=smiData.RigidTransform(8).angle  RotationAngleUnits=rad  RotationArbitraryAxis=smiData.RigidTransform(8).axis  RotationSequenceAxes=FollowerAxes  RotationSequence=XYX  RotationSequenceAngles=[0 0 0]  RotationSequenceAnglesUnits=deg  RotationMatrix=[1 0 0;0 1 0;0 0 1]  Quaternion=[1 0 0 0]  TranslationMethod=Cartesian  TranslationCartesianOffset=smiData.RigidTransform(8).translation  TranslationCartesianOffsetUnits=mm  TranslationStandardAxis=+Z  TranslationStandardOffset=0  TranslationStandardOffsetUnits=m  TranslationROffset=0  TranslationROffsetUnits=m  TranslationThetaOffset=0  TranslationThetaOffsetUnits=deg  TranslationZOffset=0  TranslationZOffsetUnits=m
  F1 : PMIOPort  Side=Left
  F : PMIOPort  Port=2  Side=Right
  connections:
  Solid/RConn1 -- ReferenceFrame/RConn1 -- Transform/LConn1 -- Transform1/LConn1
  Transform/RConn1 -- F/RConn1
  Transform1/RConn1 -- F1/RConn1

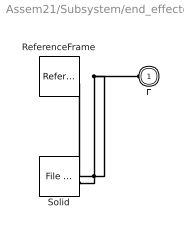
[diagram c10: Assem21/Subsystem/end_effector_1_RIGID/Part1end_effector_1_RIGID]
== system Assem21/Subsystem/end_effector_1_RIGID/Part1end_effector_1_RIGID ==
  ReferenceFrame : sm_lib/Frames and Transforms/Reference Frame
  Solid : sm_lib/Body Elements/File Solid  ExtGeomFileName=Part1-end effector_Default_sldprt.STEP  UnitType=FromFile  ExtGeomFileUnits=m  StepReaderType=HEX  ExportConvexHullGeometry=off  InertiaType=Custom  BasedOnType=DensityFromFile  Density=1000  DensityUnits=kg/m^3  Mass=smiData.Solid(4).mass  MassUnits=kg  CenterOfMass=smiData.Solid(4).CoM  CenterOfMassUnits=mm  MomentsOfInertia=smiData.Solid(4).MoI  MomentsOfInertiaUnits=kg*mm^2  ProductsOfInertia=smiData.Solid(4).PoI  ProductsOfInertiaUnits=kg*mm^2  GraphicType=FromGeometry  MarkerShape=Sphere  MarkerSize=10  GraphicVisPropType=SimpleVisualProperties  GraphicDiffuseColor=smiData.Solid(4).color  GraphicOpacity=smiData.Solid(4).opacity  GraphicSpecularColor=[0.5 0.5 0.5 1.0]  GraphicAmbientColor=[0.15 0.15 0.15 1.0]  GraphicEmissiveColor=[0.0 0.0 0.0 1.0]  GraphicShininess=75  DoExposeReferenceFrame=on  SerializedFrames=<Frames/>
  F : PMIOPort  Side=Left
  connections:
  Solid/RConn1 -- ReferenceFrame/RConn1 -- F/RConn1

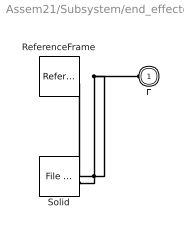
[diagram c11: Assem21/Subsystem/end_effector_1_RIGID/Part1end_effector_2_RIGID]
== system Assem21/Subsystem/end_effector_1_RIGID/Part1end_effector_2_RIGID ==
  ReferenceFrame : sm_lib/Frames and Transforms/Reference Frame
  Solid : sm_lib/Body Elements/File Solid  ExtGeomFileName=Part1-end effector_Default_sldprt.STEP  UnitType=FromFile  ExtGeomFileUnits=m  StepReaderType=HEX  ExportConvexHullGeometry=off  InertiaType=Custom  BasedOnType=DensityFromFile  Density=1000  DensityUnits=kg/m^3  Mass=smiData.Solid(4).mass  MassUnits=kg  CenterOfMass=smiData.Solid(4).CoM  CenterOfMassUnits=mm  MomentsOfInertia=smiData.Solid(4).MoI  MomentsOfInertiaUnits=kg*mm^2  ProductsOfInertia=smiData.Solid(4).PoI  ProductsOfInertiaUnits=kg*mm^2  GraphicType=FromGeometry  MarkerShape=Sphere  MarkerSize=10  GraphicVisPropType=SimpleVisualProperties  GraphicDiffuseColor=smiData.Solid(4).color  GraphicOpacity=smiData.Solid(4).opacity  GraphicSpecularColor=[0.5 0.5 0.5 1.0]  GraphicAmbientColor=[0.15 0.15 0.15 1.0]  GraphicEmissiveColor=[0.0 0.0 0.0 1.0]  GraphicShininess=75  DoExposeReferenceFrame=on  SerializedFrames=<Frames/>
  F : PMIOPort  Side=Left
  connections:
  Solid/RConn1 -- ReferenceFrame/RConn1 -- F/RConn1

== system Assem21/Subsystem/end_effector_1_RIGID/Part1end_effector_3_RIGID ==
  ReferenceFrame : sm_lib/Frames and Transforms/Reference Frame
  Solid : sm_lib/Body Elements/File Solid  ExtGeomFileName=Part1-end effector_Default_sldprt.STEP  UnitType=FromFile  ExtGeomFileUnits=m  StepReaderType=HEX  ExportConvexHullGeometry=off  InertiaType=Custom  BasedOnType=DensityFromFile  Density=1000  DensityUnits=kg/m^3  Mass=smiData.Solid(4).mass  MassUnits=kg  CenterOfMass=smiData.Solid(4).CoM  CenterOfMassUnits=mm  MomentsOfInertia=smiData.Solid(4).MoI  MomentsOfInertiaUnits=kg*mm^2  ProductsOfInertia=smiData.Solid(4).PoI  ProductsOfInertiaUnits=kg*mm^2  GraphicType=FromGeometry  MarkerShape=Sphere  MarkerSize=10  GraphicVisPropType=SimpleVisualProperties  GraphicDiffuseColor=smiData.Solid(4).color  GraphicOpacity=smiData.Solid(4).opacity  GraphicSpecularColor=[0.5 0.5 0.5 1.0]  GraphicAmbientColor=[0.15 0.15 0.15 1.0]  GraphicEmissiveColor=[0.0 0.0 0.0 1.0]  GraphicShininess=75  DoExposeReferenceFrame=on  SerializedFrames=<Frames/>
  F : PMIOPort  Side=Left
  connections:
  Solid/RConn1 -- ReferenceFrame/RConn1 -- F/RConn1

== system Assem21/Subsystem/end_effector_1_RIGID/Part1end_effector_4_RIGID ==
  ReferenceFrame : sm_lib/Frames and Transforms/Reference Frame
  Solid : sm_lib/Body Elements/File Solid  ExtGeomFileName=Part1-end effector_Default_sldprt.STEP  UnitType=FromFile  ExtGeomFileUnits=m  StepReaderType=HEX  ExportConvexHullGeometry=off  InertiaType=Custom  BasedOnType=DensityFromFile  Density=1000  DensityUnits=kg/m^3  Mass=smiData.Solid(4).mass  MassUnits=kg  CenterOfMass=smiData.Solid(4).CoM  CenterOfMassUnits=mm  MomentsOfInertia=smiData.Solid(4).MoI  MomentsOfInertiaUnits=kg*mm^2  ProductsOfInertia=smiData.Solid(4).PoI  ProductsOfInertiaUnits=kg*mm^2  GraphicType=FromGeometry  MarkerShape=Sphere  MarkerSize=10  GraphicVisPropType=SimpleVisualProperties  GraphicDiffuseColor=smiData.Solid(4).color  GraphicOpacity=smiData.Solid(4).opacity  GraphicSpecularColor=[0.5 0.5 0.5 1.0]  GraphicAmbientColor=[0.15 0.15 0.15 1.0]  GraphicEmissiveColor=[0.0 0.0 0.0 1.0]  GraphicShininess=75  DoExposeReferenceFrame=on  SerializedFrames=<Frames/>
  F : PMIOPort  Side=Left
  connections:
  Solid/RConn1 -- ReferenceFrame/RConn1 -- F/RConn1

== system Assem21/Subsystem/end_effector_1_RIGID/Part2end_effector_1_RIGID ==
  ReferenceFrame : sm_lib/Frames and Transforms/Reference Frame
  Solid : sm_lib/Body Elements/File Solid  ExtGeomFileName=Part2-end effector_Default_sldprt.STEP  UnitType=FromFile  ExtGeomFileUnits=m  StepReaderType=HEX  ExportConvexHullGeometry=off  InertiaType=Custom  BasedOnType=DensityFromFile  Density=1000  DensityUnits=kg/m^3  Mass=smiData.Solid(5).mass  MassUnits=kg  CenterOfMass=smiData.Solid(5).CoM  CenterOfMassUnits=mm  MomentsOfInertia=smiData.Solid(5).MoI  MomentsOfInertiaUnits=kg*mm^2  ProductsOfInertia=smiData.Solid(5).PoI  ProductsOfInertiaUnits=kg*mm^2  GraphicType=FromGeometry  MarkerShape=Sphere  MarkerSize=10  GraphicVisPropType=SimpleVisualProperties  GraphicDiffuseColor=smiData.Solid(5).color  GraphicOpacity=smiData.Solid(5).opacity  GraphicSpecularColor=[0.5 0.5 0.5 1.0]  GraphicAmbientColor=[0.15 0.15 0.15 1.0]  GraphicEmissiveColor=[0.0 0.0 0.0 1.0]  GraphicShininess=75  DoExposeReferenceFrame=on  SerializedFrames=<Frames/>
  F : PMIOPort  Side=Left
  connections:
  Solid/RConn1 -- ReferenceFrame/RConn1 -- F/RConn1

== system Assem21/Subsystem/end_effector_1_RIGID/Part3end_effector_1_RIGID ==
  ReferenceFrame : sm_lib/Frames and Transforms/Reference Frame
  Solid : sm_lib/Body Elements/File Solid  ExtGeomFileName=Part3-end effector_Default_sldprt.STEP  UnitType=FromFile  ExtGeomFileUnits=m  StepReaderType=HEX  ExportConvexHullGeometry=off  InertiaType=Custom  BasedOnType=DensityFromFile  Density=1000  DensityUnits=kg/m^3  Mass=smiData.Solid(6).mass  MassUnits=kg  CenterOfMass=smiData.Solid(6).CoM  CenterOfMassUnits=mm  MomentsOfInertia=smiData.Solid(6).MoI  MomentsOfInertiaUnits=kg*mm^2  ProductsOfInertia=smiData.Solid(6).PoI  ProductsOfInertiaUnits=kg*mm^2  GraphicType=FromGeometry  MarkerShape=Sphere  MarkerSize=10  GraphicVisPropType=SimpleVisualProperties  GraphicDiffuseColor=smiData.Solid(6).color  GraphicOpacity=smiData.Solid(6).opacity  GraphicSpecularColor=[0.5 0.5 0.5 1.0]  GraphicAmbientColor=[0.15 0.15 0.15 1.0]  GraphicEmissiveColor=[0.0 0.0 0.0 1.0]  GraphicShininess=75  DoExposeReferenceFrame=on  SerializedFrames=<Frames/>
  F : PMIOPort  Side=Left
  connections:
  Solid/RConn1 -- ReferenceFrame/RConn1 -- F/RConn1

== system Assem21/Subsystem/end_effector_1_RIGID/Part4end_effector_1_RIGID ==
  ReferenceFrame : sm_lib/Frames and Transforms/Reference Frame
  Solid : sm_lib/Body Elements/File Solid  ExtGeomFileName=Part4-end effector_Default_sldprt.STEP  UnitType=FromFile  ExtGeomFileUnits=m  StepReaderType=HEX  ExportConvexHullGeometry=off  InertiaType=Custom  BasedOnType=DensityFromFile  Density=1000  DensityUnits=kg/m^3  Mass=smiData.Solid(7).mass  MassUnits=kg  CenterOfMass=smiData.Solid(7).CoM  CenterOfMassUnits=mm  MomentsOfInertia=smiData.Solid(7).MoI  MomentsOfInertiaUnits=kg*mm^2  ProductsOfInertia=smiData.Solid(7).PoI  ProductsOfInertiaUnits=kg*mm^2  GraphicType=FromGeometry  MarkerShape=Sphere  MarkerSize=10  GraphicVisPropType=SimpleVisualProperties  GraphicDiffuseColor=smiData.Solid(7).color  GraphicOpacity=smiData.Solid(7).opacity  GraphicSpecularColor=[0.5 0.5 0.5 1.0]  GraphicAmbientColor=[0.15 0.15 0.15 1.0]  GraphicEmissiveColor=[0.0 0.0 0.0 1.0]  GraphicShininess=75  DoExposeReferenceFrame=on  SerializedFrames=<Frames/>
  F : PMIOPort  Side=Left
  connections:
  Solid/RConn1 -- ReferenceFrame/RConn1 -- F/RConn1

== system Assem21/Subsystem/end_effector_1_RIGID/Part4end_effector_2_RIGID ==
  ReferenceFrame : sm_lib/Frames and Transforms/Reference Frame
  Solid : sm_lib/Body Elements/File Solid  ExtGeomFileName=Part4-end effector_Default_sldprt.STEP  UnitType=FromFile  ExtGeomFileUnits=m  StepReaderType=HEX  ExportConvexHullGeometry=off  InertiaType=Custom  BasedOnType=DensityFromFile  Density=1000  DensityUnits=kg/m^3  Mass=smiData.Solid(7).mass  MassUnits=kg  CenterOfMass=smiData.Solid(7).CoM  CenterOfMassUnits=mm  MomentsOfInertia=smiData.Solid(7).MoI  MomentsOfInertiaUnits=kg*mm^2  ProductsOfInertia=smiData.Solid(7).PoI  ProductsOfInertiaUnits=kg*mm^2  GraphicType=FromGeometry  MarkerShape=Sphere  MarkerSize=10  GraphicVisPropType=SimpleVisualProperties  GraphicDiffuseColor=smiData.Solid(7).color  GraphicOpacity=smiData.Solid(7).opacity  GraphicSpecularColor=[0.5 0.5 0.5 1.0]  GraphicAmbientColor=[0.15 0.15 0.15 1.0]  GraphicEmissiveColor=[0.0 0.0 0.0 1.0]  GraphicShininess=75  DoExposeReferenceFrame=on  SerializedFrames=<Frames/>
  F : PMIOPort  Side=Left
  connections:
  Solid/RConn1 -- ReferenceFrame/RConn1 -- F/RConn1

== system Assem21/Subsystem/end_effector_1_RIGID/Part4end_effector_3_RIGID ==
  ReferenceFrame : sm_lib/Frames and Transforms/Reference Frame
  Solid : sm_lib/Body Elements/File Solid  ExtGeomFileName=Part4-end effector_Default_sldprt.STEP  UnitType=FromFile  ExtGeomFileUnits=m  StepReaderType=HEX  ExportConvexHullGeometry=off  InertiaType=Custom  BasedOnType=DensityFromFile  Density=1000  DensityUnits=kg/m^3  Mass=smiData.Solid(7).mass  MassUnits=kg  CenterOfMass=smiData.Solid(7).CoM  CenterOfMassUnits=mm  MomentsOfInertia=smiData.Solid(7).MoI  MomentsOfInertiaUnits=kg*mm^2  ProductsOfInertia=smiData.Solid(7).PoI  ProductsOfInertiaUnits=kg*mm^2  GraphicType=FromGeometry  MarkerShape=Sphere  MarkerSize=10  GraphicVisPropType=SimpleVisualProperties  GraphicDiffuseColor=smiData.Solid(7).color  GraphicOpacity=smiData.Solid(7).opacity  GraphicSpecularColor=[0.5 0.5 0.5 1.0]  GraphicAmbientColor=[0.15 0.15 0.15 1.0]  GraphicEmissiveColor=[0.0 0.0 0.0 1.0]  GraphicShininess=75  DoExposeReferenceFrame=on  SerializedFrames=<Frames/>
  F : PMIOPort  Side=Left
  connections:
  Solid/RConn1 -- ReferenceFrame/RConn1 -- F/RConn1
